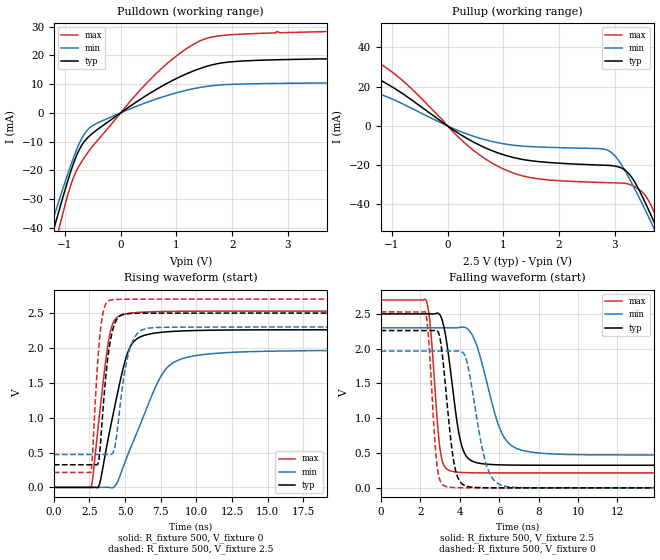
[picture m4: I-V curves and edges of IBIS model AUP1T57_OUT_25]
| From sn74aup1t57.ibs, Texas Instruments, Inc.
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[Model]   AUP1T57_OUT_25
Model_type  Output
Vref =   0
Rref =   1E6
Cref =   30p
Vmeas =   1.25
| variable   typ   min   max
C_comp   2.77pF   1.87pF   4.14pF
| C_pullup   3.12pF   1.87pF   4.14pF
| C_pulldown   2.42pF   2.13pF   2.99pF
[Temperature Range]   40   100   -40
| Ambient temperature   25   85   -40
[Voltage range]   2.5   2.3   2.7
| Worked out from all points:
|   slope of the pulldown table from 0 to 0.375 V, typ, clamps not added: 75.2 ohm
|   slope of the pullup table from 0 to 0.375 V, typ, clamps not added: 55.1 ohm
|   rising waveform, R_fixture 500, V_fixture 0: 20-80 % time 1.4ns typ, 2.41ns min, 858ps max; typ from 0 V to 2.26 V
|   falling waveform, R_fixture 500, V_fixture 2.5: 20-80 % time 622ps typ, 1.07ns min, 391ps max; typ from 2.5 V to 0.325 V
|   rising waveform, R_fixture 500, V_fixture 2.5: 20-80 % time 612ps typ, 791ps min, 470ps max; typ from 0.325 V to 2.5 V
|   falling waveform, R_fixture 500, V_fixture 0: 20-80 % time 497ps typ, 751ps min, 332ps max; typ from 2.26 V to 0 V
[Pulldown]
| AUP1T57_OUT_25
|   Voltage   I(typ)   I(min)   I(max)
-3.6V     -214mA     -193.5mA   -239.7mA
-1.26V    -44.55mA   -39.92mA   -52.42mA
-1.205V   -40.74mA   -36.52mA   -48.02mA
-1.115V   -34.57mA   -31.02mA   -40.91mA
-800mV    -15.22mA   -13.22mA   -20.4mA
-685mV    -10.84mA   -8.445mA   -16.54mA
-540mV    -7.689mA   -4.911mA   -12.5mA
675mV     8.558mA    5.038mA    14.35mA
1.105V    12.9mA     7.5mA      21.28mA
1.52V     16.03mA    9.129mA    25.76mA
2.585V    18.34mA    10.19mA    27.69mA
7.2V      19.61mA    10.73mA    29.61mA
[Pullup]
| AUP1T57_OUT_25
|   Voltage   I(typ)   I(min)   I(max)
-3.6V     37.28mA    23.5mA     50.35mA
-2.355V   24.65mA    15.21mA    35.57mA
-1.425V   26.01mA    17.2mA     35.58mA
-760mV    15.58mA    10.63mA    21.96mA
405mV     -7.279mA   -4.651mA   -11.04mA
1.05V     -15.07mA   -9.293mA   -22.54mA
2.845V    -20.04mA   -12.07mA   -28.88mA
3.17V     -22.17mA   -22.09mA   -29.2mA
3.455V    -33.67mA   -37.48mA   -32.73mA
3.685V    -47.61mA   -50.92mA   -42.5mA
3.82V     -56.28mA   -59.04mA   -51.47mA
7.2V      -294.7mA   -278.7mA   -311.5mA
[Ramp]
| AUP1T57_OUT_25
| variable   typ   min   max
dV/dt_r   1.36/1.41E-09   1.18/2.41E-09   1.52/8.59E-10
dV/dt_f   1.31/6.27E-10   1.10/1.07E-09   1.50/3.94E-10
R_load = 500
[Rising Waveform]
| AUP1T57_OUT_25
R_fixture =   500
C_fixture =   0
L_fixture =   0
V_fixture =   0
V_fixture_min = 0
V_fixture_max = 0
|   Time   V(typ)   V(min)   V(max)
0s        19.04nV    76.96nV    1.464nV
2.615ns   1.81uV     23.81nV    1.836mV
3.19ns    38.12mV    731.8nV    1.014V
3.875ns   761.3mV    -61.17uV   2.14V
4.75ns    1.61V      226.5mV    2.471V
5.26ns    1.972V     503.4mV    2.495V
5.825ns   2.13V      782.3mV    2.508V
7.615ns   2.226V     1.628V     2.522V
9.17ns    2.245V     1.856V     2.526V
34.99ns   2.261V     1.966V     2.528V
[Falling Waveform]
| AUP1T57_OUT_25
R_fixture =   500
C_fixture =   0
L_fixture =   0
V_fixture =   2.5
V_fixture_min = 2.3
V_fixture_max = 2.7
|   Time   V(typ)   V(min)   V(max)
0s        2.5V       2.3V       2.7V
2.315ns   2.5V       2.3V       2.686V
2.525ns   2.5V       2.3V       2.293V
3.02ns    2.477V     2.3V       532.2mV
3.605ns   1.531V     2.299V     238.1mV
4ns       730.2mV    2.305V     222.9mV
4.395ns   435.7mV    2.287V     217.9mV
6.13ns    329.9mV    793.1mV    214.5mV
7.355ns   325.9mV    527.4mV    214.4mV
34.99ns   324.7mV    472mV      214.4mV
[Rising Waveform]
| AUP1T57_OUT_25
R_fixture =   500
C_fixture =   0
L_fixture =   0
V_fixture =   2.5
V_fixture_min = 2.3
V_fixture_max = 2.7
|   Time   V(typ)   V(min)   V(max)
0s        324.7mV    472mV      214.4mV
2.605ns   324.7mV    472mV      218.5mV
3.075ns   329.6mV    472mV      1.784V
3.26ns    592.7mV    471.9mV    2.231V
3.54ns    1.345V     472.2mV    2.574V
3.925ns   2.054V     471.3mV    2.683V
4.305ns   2.365V     602.7mV    2.694V
5.28ns    2.493V     1.951V     2.698V
6.395ns   2.498V     2.274V     2.699V
34.99ns   2.5V       2.3V       2.7V
[Falling Waveform]
| AUP1T57_OUT_25
R_fixture =   500
C_fixture =   0
L_fixture =   0
V_fixture =   0
V_fixture_min = 0
V_fixture_max = 0
|   Time   V(typ)   V(min)   V(max)
0s        2.261V     1.966V     2.528V
2.275ns   2.261V     1.966V     2.515V
2.85ns    2.261V     1.966V     335mV
3.315ns   1.37V      1.966V     18.59mV
3.665ns   444.1mV    1.966V     5.514mV
3.995ns   99.8mV     1.966V     1.957mV
4.39ns    20.67mV    1.79V      603.1uV
5.385ns   1.305mV    305.9mV    52.28uV
6.295ns   218.2uV    24.08mV    8.998uV
34.99ns   -10.73nV   66.69nV    -18.87nV
